[IBIS Ver]   3.2
[File Name]   lm3s2950_bga_v0p1.ibs
[File Rev]   0.1
[Date]   02/19/2010
[Source]   From silicon level SPICE simulations at Texas Instruments
[Notes]   Initial Release of IBIS model
   LM3S2950, Revision A2, 108 BGA
[Disclaimer] Texas Instruments Confidential - Advance Product Information
   < Software License Agreement >
  Texas Instruments (TI) is supplying this software for use solely and
  exclusively on TI's Stellaris Family of microcontroller products.
  The software is owned by TI and/or its suppliers, and is protected under
  applicable copyright laws.  All rights are reserved.  Any use in violation
  of the foregoing restrictions may subject the user to criminal sanctions
  under applicable laws, as well as to civil liability for the breach of the
  terms and conditions of this license.
  THIS SOFTWARE IS PROVIDED "AS IS".  NO WARRANTIES, WHETHER EXPRESS, IMPLIED
  OR STATUTORY, INCLUDING, BUT NOT LIMITED TO, IMPLIED WARRANTIES OF
  MERCHANTABILITY AND FITNESS FOR A PARTICULAR PURPOSE APPLY TO THIS SOFTWARE.
  LMI SHALL NOT, IN ANY CIRCUMSTANCES, BE LIABLE FOR SPECIAL, INCIDENTAL, OR
  CONSEQUENTIAL DAMAGES, FOR ANY REASON WHATSOEVER.
[Copyright]   Copyright (c) 2010 Texas Instruments.  All rights reserved.
[Component]   LM3S2950 108BGA
[Manufacturer]  Texas Instruments
[Package]
| 108-pin BGA
| variable   typ   min   max
R_pkg   84.738m   52.939m   202.980m
L_pkg   2.011nH   1.073nH   6.026nH
C_pkg   0.754pF   0.419pF   1.686pF
[Pin]  signal_name   model_name   R_pin   L_pin   C_pin
  A1   NC   NC   79.888m   1.323nH   0.715pF
  A2   NC   NC   90.104m   1.724nH   0.912pF
  A3   NC   NC   98.401m   1.913nH   1.194pF
  A4   NC   NC   87.067m   1.486nH   1.215pF
  A5   GNDA   GND   96.822m   3.026nH   0.689pF
  A6   PB4   ProgBuff1   95.630m   1.938nH   0.455pF
  A7   PB6   ProgBuff1   101.890m   2.158nH   0.497pF
  A8   PB7_TRST   ProgBuff1   104.270m   2.377nH   0.515pF
  A9   PC0_TCK_SWCLK   ProgBuff1   84.760m   1.452nH   0.421pF
 A10   PC3_TDO_SWO   ProgBuff1   99.044m   1.987nH   0.424pF
 A11   PE0_SSI1Clk   ProgBuff1   113.360m   2.943nH   0.668pF
 A12   PE3_SSI1Tx   ProgBuff1   101.080m   2.474nH   0.511pF
  B1   NC   NC   87.244m   1.692nH   0.517pF
  B2   NC   NC   81.244m   1.515nH   0.770pF
  B3   NC   NC   80.154m   1.140nH   0.800pF
  B4   NC   NC   79.328m   1.173nH   1.161pF
  B5   GNDA   GND   96.822m   3.026nH   0.689pF
  B6   GND   GND   58.071m   1.495nH   1.068pF
  B7   PB5   ProgBuff1   95.103m   2.064nH   0.608pF
  B8   PC2_TDI   ProgBuff1   119.340m   2.620nH   0.599pF
  B9   PC1_TMS_SWDIO   ProgBuff1   80.684m   1.224nH   0.423pF
 B10   CMOD1   NC   87.340m   1.384nH   0.448pF
 B11   PE2_SSI1Rx   ProgBuff1   102.350m   2.101nH   0.494pF
 B12   PE1_SSI1Fss   ProgBuff1   94.086m   2.106nH   0.459pF
  C1   PE7_PWM5   ProgBuff0   87.244m   1.692nH   0.517pF
  C2   PE6_PWM4   ProgBuff0   79.888m   1.323nH   0.715pF
  C3   VDD25   POWER   95.640m   3.704nH   1.367pF
  C4   GND   GND   58.071m   1.495nH   1.068pF
  C5   GND   GND   58.071m   1.495nH   1.068pF
  C6   VDDA   POWER   100.856m   3.274nH   0.728pF
  C7   VDDA   POWER   100.856m   3.274nH   0.728pF
  C8   PH1_PWM3   ProgBuff2   94.132m   1.905nH   0.651pF
  C9   PH0_PWM2   ProgBuff2   104.080m   2.081nH   0.818pF
 C10   PG7   ProgBuff2   202.980m   6.026nH   1.686pF
 C11   PB2_I2C0SCL   ProgBuff1   56.199m   1.699nH   0.640pF
 C12   PB3_I2C0SDA   ProgBuff1   92.913m   2.095nH   0.464pF
  D1   PE4   ProgBuff0   81.244m   1.515nH   0.770pF
  D2   PE5_CCP5   ProgBuff0   80.154m   1.140nH   0.800pF
  D3   VDD25   POWER   95.640m   3.704nH   1.367pF
 D10   PH3_PhB0   ProgBuff2   108.850m   2.225nH   0.869pF
 D11   PH2   ProgBuff2   140.460m   3.016nH   0.999pF
 D12   PB1_CCP2   ProgBuff1   103.650m   2.276nH   0.565pF
  E1   PD4_CCP3   ProgBuff0   87.067m   1.486nH   1.215pF
  E2   PD5   ProgBuff0   79.328m   1.173nH   1.161pF
  E3   LDO   POWER   52.939m   1.073nH   0.655pF
 E10   VDD33   POWER   66.656m   2.704nH   1.051pF
 E11   CMOD0   NC   91.511m   1.493nH   0.644pF
 E12   PB0_CCP0   ProgBuff1   94.165m   1.998nH   0.486pF
  F1   PD7_IDX0   ProgBuff0   90.104m   1.724nH   0.912pF
  F2   PD6_Fault   ProgBuff0   98.401m   1.913nH   1.194pF
  F3   VDD25   POWER   95.640m   3.704nH   1.367pF
 F10   GND   GND   58.071m   1.495nH   1.068pF
 F11   GND   GND   58.071m   1.495nH   1.068pF
 F12   GND   GND   58.071m   1.495nH   1.068pF
  G1   PD0_CAN0Rx   ProgBuff1   92.619m   1.798nH   0.474pF
  G2   PD1_CAN0Tx   ProgBuff1   79.925m   1.248nH   0.494pF
  G3   VDD25   POWER   95.640m   3.704nH   1.367pF
 G10   VDD33   POWER   66.656m   2.704nH   1.051pF
 G11   VDD33   POWER   66.656m   2.704nH   1.051pF
 G12   VDD33   POWER   66.656m   2.704nH   1.051pF
  H1   PD3_U1Tx   ProgBuff1   99.883m   1.949nH   0.529pF
  H2   PD2_U1Rx   ProgBuff1   88.523m   1.653nH   0.586pF
  H3   GND   GND   58.071m   1.495nH   1.068pF
 H10   VDD33   POWER   66.656m   2.704nH   1.051pF
 H11   RST   NC   83.383m   1.433nH   0.517pF
 H12   PF1_CAN1Tx   ProgBuff1   93.021m   1.786nH   0.467pF
  J1   PG2_PWM0   ProgBuff2   96.583m   2.036nH   0.496pF
  J2   PG3_PWM1   ProgBuff2   89.912m   1.491nH   0.627pF
  J3   GND   GND   58.071m   1.495nH   1.068pF
 J10   GND   GND   58.071m   1.495nH   1.068pF
 J11   PF2   ProgBuff1   89.129m   1.622nH   0.584pF
 J12   PF3   ProgBuff1   101.960m   2.118nH   0.517pF
  K1   PG0_U2Rx   ProgBuff1   102.390m   2.208nH   0.502pF
  K2   PG1_U2Tx   ProgBuff1   100.800m   2.153nH   0.623pF
  K3   PG4   ProgBuff2   154.100m   3.393nH   1.099pF
  K4   PF7   ProgBuff2   124.990m   2.888nH   0.991pF
  K5   GND   GND   58.071m   1.495nH   1.068pF
  K6   GND   GND   58.071m   1.495nH   1.068pF
  K7   VDD33   POWER   66.656m   2.704nH   1.051pF
  K8   VDD33   POWER   66.656m   2.704nH   1.051pF
  K9   VDD33   POWER   66.656m   2.704nH   1.051pF
 K10   GND   GND   58.071m   1.495nH   1.068pF
 K11   XOSC0   NC   86.559m   1.259nH   0.607pF
 K12   XOSC1   NC   86.113m   1.460nH   0.432pF
  L1   PC4_PhA0   ProgBuff1   98.609m   2.032nH   0.480pF
  L2   PC7   ProgBuff1   92.556m   1.569nH   0.579pF
  L3   PA0_U0Rx   ProgBuff1   87.729m   1.568nH   0.451pF
  L4   PA3_SSI0Fss   ProgBuff1   92.956m   1.603nH   0.522pF
  L5   PA4_SSI0Rx   ProgBuff1   90.643m   1.244nH   0.596pF
  L6   PA6_CCP1   ProgBuff1   84.555m   1.313nH   0.460pF
  L7   PG6   ProgBuff2   77.821m   1.124nH   0.483pF
  L8   PF5_C1o   ProgBuff2   79.888m   1.306nH   0.515pF
  L9   PF4_C0o   ProgBuff1   115.890m   2.346nH   0.895pF
 L10   GND   GND   58.071m   1.495nH   1.068pF
 L11   OSC0   NC   89.148m   1.889nH   0.583pF
 L12   VBAT   POWER   96.383m   2.176nH   0.477pF
  M1   PC5   ProgBuff1   104.060m   2.479nH   0.492pF
  M2   PC6   ProgBuff1   106.250m   2.417nH   0.544pF
  M3   PA1_U0Tx   ProgBuff1   102.070m   2.145nH   0.473pF
  M4   PA2_SSI0Clk   ProgBuff1   105.080m   2.043nH   0.432pF
  M5   PA5_SSI0Tx   ProgBuff1   99.089m   1.878nH   0.481pF
  M6   PA7_CCP4   ProgBuff1   91.460m   1.784nH   0.458pF
  M7   PG5   ProgBuff2   84.574m   1.455nH   0.457pF
  M8   PF6_C2o   ProgBuff2   92.410m   1.707nH   0.460pF
  M9   PF0_CAN1Rx   ProgBuff1   88.587m   1.632nH   0.419pF
 M10   WAKE   NC   84.093m   1.457nH   0.453pF
 M11   OSC1   NC   93.495m   2.102nH   0.500pF
 M12   HIB   NC   102.740m   2.327nH   0.492pF
[Package Model]   TI-108-BGA-01108004-1
[Model Selector]   ProgBuff0
I/O_2_0   2 mA buffer without slew rate control
I/O_4_0   4 mA buffer without slew rate control
I/O_8_0   8 mA buffer without slew rate control
I/O_8S_0   8 mA buffer with slew rate control
OD_I/O_2_0   open-drain 2 mA buffer without slew rate control
OD_I/O_4_0   open-drain 4 mA buffer without slew rate control
OD_I/O_8_0   open-drain 8 mA buffer without slew rate control
OD_I/O_8S_0   open-drain 8 mA buffer with slew rate control
WPU_I/O_2_0   weak pullup 2 mA buffer without slew rate control
WPU_I/O_4_0   weak pullup 4 mA buffer without slew rate control
WPU_I/O_8_0   weak pullup 8 mA buffer without slew rate control
WPU_I/O_8S_0   weak pullup 8 mA buffer with slew rate control
WPD_I/O_2_0   weak pulldown 2 mA buffer without slew rate control
WPD_I/O_4_0   weak pulldown 4 mA buffer without slew rate control
WPD_I/O_8_0   weak pulldown 8 mA buffer without slew rate control
WPD_I/O_8S_0   weak pulldown 8 mA buffer with slew rate control
[Model Selector]   ProgBuff1
I/O_2_1   2 mA buffer without slew rate control
I/O_4_1   4 mA buffer without slew rate control
I/O_8_1   8 mA buffer without slew rate control
I/O_8S_1   8 mA buffer with slew rate control
OD_I/O_2_1   open-drain 2 mA buffer without slew rate control
OD_I/O_4_1   open-drain 4 mA buffer without slew rate control
OD_I/O_8_1   open-drain 8 mA buffer without slew rate control
OD_I/O_8S_1   open-drain 8 mA buffer with slew rate control
WPU_I/O_2_1   weak pullup 2 mA buffer without slew rate control
WPU_I/O_4_1   weak pullup 4 mA buffer without slew rate control
WPU_I/O_8_1   weak pullup 8 mA buffer without slew rate control
WPU_I/O_8S_1   weak pullup 8 mA buffer with slew rate control
WPD_I/O_2_1   weak pulldown 2 mA buffer without slew rate control
WPD_I/O_4_1   weak pulldown 4 mA buffer without slew rate control
WPD_I/O_8_1   weak pulldown 8 mA buffer without slew rate control
WPD_I/O_8S_1   weak pulldown 8 mA buffer with slew rate control
[Model Selector]   ProgBuff2
I/O_2_2   2 mA buffer without slew rate control
I/O_4_2   4 mA buffer without slew rate control
I/O_8_2   8 mA buffer without slew rate control
I/O_8S_2   8 mA buffer with slew rate control
OD_I/O_2_2   open-drain 2 mA buffer without slew rate control
OD_I/O_4_2   open-drain 4 mA buffer without slew rate control
OD_I/O_8_2   open-drain 8 mA buffer without slew rate control
OD_I/O_8S_2   open-drain 8 mA buffer with slew rate control
WPU_I/O_2_2   weak pullup 2 mA buffer without slew rate control
WPU_I/O_4_2   weak pullup 4 mA buffer without slew rate control
WPU_I/O_8_2   weak pullup 8 mA buffer without slew rate control
WPU_I/O_8S_2   weak pullup 8 mA buffer with slew rate control
WPD_I/O_2_2   weak pulldown 2 mA buffer without slew rate control
WPD_I/O_4_2   weak pulldown 4 mA buffer without slew rate control
WPD_I/O_8_2   weak pulldown 8 mA buffer without slew rate control
WPD_I/O_8S_2   weak pulldown 8 mA buffer with slew rate control
[Define Package Model]  TI-108-BGA-01108004-1
[Manufacturer]   Texas Instruments, Inc.
[OEM]   ASAT Holdings Limited
[Description]   TI 108 Ball Grid Array package
[Number Of Pins]   108
[Pin Numbers]
A1
A2
A3
A4
A5
A6
A7
A8
A9
A10
A11
A12
B1
B2
B3
B4
B5
B6
B7
B8
B9
B10
B11
B12
C1
C2
C3
C4
C5
C6
C7
C8
C9
C10
C11
C12
D1
D2
D3
D10
D11
D12
E1
E2
E3
E10
E11
E12
F1
F2
F3
F10
F11
F12
G1
G2
G3
G10
G11
G12
H1
H2
H3
H10
H11
H12
J1
J2
J3
J10
J11
J12
K1
K2
K3
K4
K5
K6
K7
K8
K9
K10
K11
K12
L1
L2
L3
L4
L5
L6
L7
L8
L9
L10
L11
L12
M1
M2
M3
M4
M5
M6
M7
M8
M9
M10
M11
M12
[Model Data]
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[End Model Data]
[End Package Model]
| Models and submodels in the file (48): I/O_2_0 (I/O), I/O_4_0 (I/O), I/O_8_0 (I/O), I/O_8S_0 (I/O), OD_I/O_2_0 (I/O_open_drain), OD_I/O_4_0 (I/O_open_drain), OD_I/O_8_0 (I/O_open_drain), OD_I/O_8S_0 (I/O_open_drain), WPU_I/O_2_0 (I/O), WPU_I/O_4_0 (I/O), WPU_I/O_8_0 (I/O), WPU_I/O_8S_0 (I/O), WPD_I/O_2_0 (I/O), WPD_I/O_4_0 (I/O), WPD_I/O_8_0 (I/O), WPD_I/O_8S_0 (I/O), I/O_2_1 (I/O), I/O_4_1 (I/O), I/O_8_1 (I/O), I/O_8S_1 (I/O), OD_I/O_2_1 (I/O_open_drain), OD_I/O_4_1 (I/O_open_drain), OD_I/O_8_1 (I/O_open_drain), OD_I/O_8S_1 (I/O_open_drain), WPU_I/O_2_1 (I/O), WPU_I/O_4_1 (I/O), WPU_I/O_8_1 (I/O), WPU_I/O_8S_1 (I/O), WPD_I/O_2_1 (I/O), WPD_I/O_4_1 (I/O), WPD_I/O_8_1 (I/O), WPD_I/O_8S_1 (I/O), I/O_2_2 (I/O), I/O_4_2 (I/O), I/O_8_2 (I/O), I/O_8S_2 (I/O), OD_I/O_2_2 (I/O_open_drain), OD_I/O_4_2 (I/O_open_drain), OD_I/O_8_2 (I/O_open_drain), OD_I/O_8S_2 (I/O_open_drain), WPU_I/O_2_2 (I/O), WPU_I/O_4_2 (I/O), WPU_I/O_8_2 (I/O), WPU_I/O_8S_2 (I/O), WPD_I/O_2_2 (I/O), WPD_I/O_4_2 (I/O), WPD_I/O_8_2 (I/O), WPD_I/O_8S_2 (I/O)
